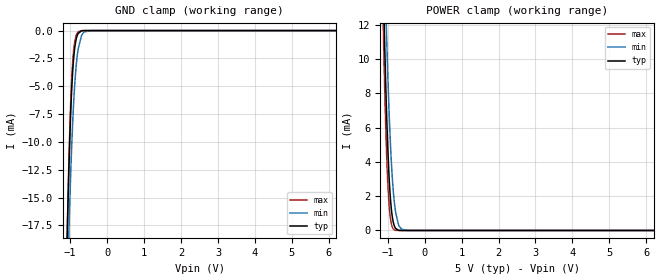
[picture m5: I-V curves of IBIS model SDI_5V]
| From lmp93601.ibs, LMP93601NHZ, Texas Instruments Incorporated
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|   Model SDI_5V
[Model]   SDI_5V
Model_type   Input
Vinl = 1.35
Vinh = 3.85
|   typ   min   max
|   (nom PVT)   (fast PVT)   (slow PVT)
C_comp   0.1436pF   0.1360pF   0.1525pF
[Model spec]
|subparameter
Vinl   1.5   1.35   1.65
Vinh   3.5   3.15   3.85
[Voltage Range]   5.0   4.5   5.5
[Temperature Range]   27   125   -25
[Power Clamp Reference]   5.0   4.5   5.5
[GND Clamp Reference]   0   0   0
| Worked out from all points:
|   GND clamp passes 1 mA (typ) near -0.85 V on its own axis
|   POWER clamp passes 1 mA (typ) near -0.89 V on its own axis
[GND Clamp]
|   Voltage   I(typ)   I(min)   I(max)
-5V       -931mA     -841.7mA   -990.9mA
-1.085V   -19.12mA   -24.53mA   -19.08mA
-1.07V    -16.98mA   -22.54mA   -16.71mA
-1.04V    -13.06mA   -18.79mA   -12.43mA
-1.025V   -11.31mA   -17.04mA   -10.55mA
-980mV    -6.906mA   -12.33mA   -5.968mA
-935mV    -3.84mA    -8.491mA   -2.991mA
-890mV    -1.94mA    -5.55mA    -1.317mA
-830mV    -668.1uA   -2.901mA   -359.3uA
-695mV    -26.7uA    -469.2uA   -7.095uA
-440mV    -371.4nA   -2.176uA   0A
9.985V    0A         0A         0A
[POWER Clamp]
|   Voltage   I(typ)   I(min)   I(max)
-5V       579.1mA    527.5mA    611.4mA
-1.13V    15.43mA    19.78mA    12.93mA
-1.115V   13.97mA    18.41mA    11.41mA
-1.085V   11.21mA    15.78mA    8.613mA
-1.04V    7.59mA     12.15mA    5.132mA
-1.01V    5.582mA    9.968mA    3.369mA
-965mV    3.248mA    7.121mA    1.579mA
-890mV    1.045mA    3.604mA    307.7uA
-800mV    173.6uA    1.289mA    18.8uA
-680mV    5.692uA    220.7uA    121.3nA
-455mV    0A         1.47uA     0A
9.985V    0A         0A         0A
